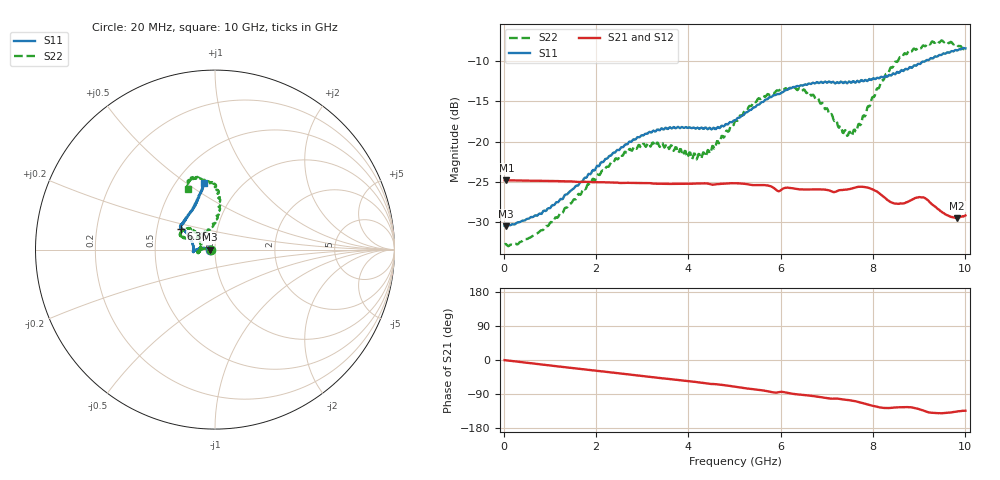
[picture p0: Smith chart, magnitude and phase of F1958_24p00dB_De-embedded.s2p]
! Integrated Device Technology
! Corporate Headquarters
! 6024 Silver Creek Valley Road
! San Jose, CA 95138  USA
! Phone:  1-408-284-8200
! Toll Free:  1-800-223-1366
! Webpage:  http://www.idt.com/
! Timing and RF Division
! 515 Groton Road, Suite 102
! Westford, MA 01886-6024
! Device:  F1958
! Description: 7-bit 0.25 dB Digital Step Attenuator
! Frequency:  0.001 -  6.000 GHz
! Package:  4x4 mm Thin QFN Plastic Package: 24 pin
! Ports:  2 RF, 12 DC
!  Pin  1  = D0
!  Pin  2  = VDD
!  Pin  3  = VMODE
!  Pin  4  = GND
!  Pin  5  = RF1  =  Port 1
!  Pin  6  = GND
!  Pin  7  = GND
!  Pin  8  = GND
!  Pin  9  = GND
!  Pin 10  = GND
!  Pin 11  = GND
!  Pin 12  = GND
!  Pin 13  = GND
!  Pin 14  = RF2  =  Port 2
!  Pin 15  = GND
!  Pin 16  = LE
!  Pin 17  = CLK
!  Pin 18  = DATA
!  Pin 19  = D6
!  Pin 20  = D5
!  Pin 21  = D4
!  Pin 22  = D3
!  Pin 23  = D2
!  Pin 24  = D1
! State:  96
! Atten State:  24.00 dB
! Voltage:  +3.30 Volts
! Current:  0.258 mA
! Data:  The device was measured on a F1958 evaluation board which has
!  individual transmission lines to the RF pins.  Data was collected
!  using a calibrated network analyzer.  The evaluation board was
!  de-embedded using Automatic Fixture Removal (AFR).
!  The reference plane is the edge of the package pin.
! Misc:
!  Action Tracker AT0419
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# GHz S dB R 50
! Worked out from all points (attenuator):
!   500 points, 20 MHz to 10 GHz, reference 50 ohm
!   highest |S21| = -24.80 dB at 60 MHz (marker M1); lowest = -29.5 dB at 9.82 GHz (marker M2)
!   lowest |S11| = -30.5 dB at 40 MHz (marker M3), VSWR 1.06, Z = 47.1 - j0.0454 ohm
!   |S11| at or under -10 dB: start of sweep to 9.137 GHz
!   |S22| runs from -33.0 to -7.5 dB; largest |S21 - S12| = 0.00031
!   S11 on the Smith chart (normalised r, x): 20 MHz: 0.94, -0.00; 6.36 GHz: 0.67, +0.16; 10 GHz: 0.67, +0.59
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0.02  -30.44 -178.9  -24.80 -0.3  -24.80 -0.3  -32.70 -178.7
0.04  -30.48 -179.1  -24.80 -0.6  -24.79 -0.6  -32.68 -178.2
0.06  -30.46 180.0  -24.80 -0.9  -24.79 -0.9  -32.75 -178.2
0.84  -28.79 171.5  -24.87 -12.1  -24.86 -12.1  -30.98 172.9
1.7  -24.97 171.8  -24.99 -24.0  -24.99 -24.0  -26.12 172.4
2.62  -20.42 177.9  -25.12 -36.8  -25.10 -36.8  -21.27 -178.5
3.36  -18.58 -174.9  -25.23 -47.3  -25.22 -47.4  -20.46 -168.4
4.24  -18.44 -178.4  -25.20 -59.2  -25.21 -59.3  -21.56 169.9
4.5  -18.50 175.7  -25.33 -63.4  -25.35 -63.4  -20.96 152.4
5.02  -17.36 161.3  -25.15 -70.6  -25.16 -70.6  -17.38 138.8
5.56  -15.25 150.7  -25.39 -79.3  -25.40 -79.3  -14.74 141.0
6.36  -13.11 148.3  -25.88 -90.7  -25.89 -90.7  -13.63 155.8
6.68  -12.77 146.7  -25.92 -94.8  -25.93 -94.7  -14.27 157.9
7.5  -12.60 138.3  -25.88 -106.3  -25.88 -106.2  -18.78 120.2
7.68  -12.56 135.4  -25.61 -110.6  -25.61 -110.5  -17.86 100.3
7.9  -12.37 128.9  -25.73 -117.9  -25.71 -117.9  -15.59 89.8
8.34  -11.77 119.0  -27.33 -126.8  -27.34 -126.9  -11.42 84.1
8.9  -10.55 109.8  -27.01 -126.7  -27.03 -126.7  -8.51 93.9
9.12  -10.09 106.4  -26.99 -134.5  -26.95 -134.6  -8.20 100.6
9.38  -9.49 103.1  -28.24 -140.3  -28.23 -140.3  -7.49 105.9
9.82  -8.72 100.4  -29.45 -136.1  -29.45 -135.7  -8.03 113.1
10  -8.46 99.7  -29.15 -133.8  -29.18 -133.8  -8.64 113.5
